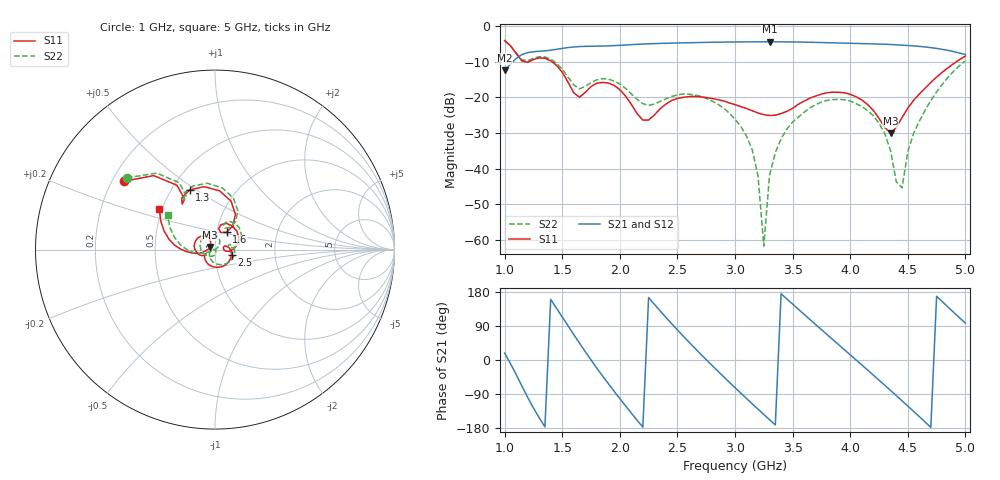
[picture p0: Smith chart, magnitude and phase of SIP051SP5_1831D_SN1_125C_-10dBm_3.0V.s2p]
# GHz  S  dB  R  50
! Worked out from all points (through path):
!   81 points, 1 GHz to 5 GHz, reference 50 ohm
!   highest |S21| = -4.32 dB at 3.3 GHz (marker M1); lowest = -12.4 dB at 1 GHz (marker M2)
!   lowest |S11| = -30.0 dB at 4.35 GHz (marker M3), VSWR 1.07, Z = 47.2 + j1.32 ohm
!   |S11| at or under -10 dB: 1.188 GHz to 1.206 GHz (18.48 MHz wide, 1.54 % of centre); 1.414 GHz to 4.919 GHz (3.506 GHz wide, 111 % of centre)
!   |S22| runs from -61.8 to -4.0 dB; largest |S21 - S12| = 0.0017
!   S11 on the Smith chart (normalised r, x): 1 GHz: 0.25, +0.31; 1.3 GHz: 0.62, +0.47; 1.6 GHz: 1.11, +0.22; 2.5 GHz: 1.20, -0.07; 5 GHz: 0.48, +0.25
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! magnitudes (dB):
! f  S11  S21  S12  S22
! 1 GHz  -4.0  -12.4  -12.4  -4.0
! 1.3 GHz  -8.8  -7.0  -7.0  -8.5
! 1.6 GHz  -18.7  -5.8  -5.8  -16.5
! 1.7 GHz  -18.6  -5.6  -5.6  -16.9
! 1.95 GHz  -16.6  -5.4  -5.4  -15.4
! 2.2 GHz  -26.4  -5.0  -5.0  -21.7
! 2.35 GHz  -23.2  -4.8  -4.8  -21.1
! 2.5 GHz  -20.3  -4.7  -4.7  -19.3
! 3 GHz  -22.0  -4.4  -4.4  -26.1
! 3.15 GHz  -23.7  -4.3  -4.3  -34.8
! 3.2 GHz  -24.4  -4.3  -4.3  -42.1
! 3.25 GHz  -24.8  -4.3  -4.3  -61.8
! 3.3 GHz  -25.1  -4.3  -4.3  -41.8
! 3.45 GHz  -23.9  -4.4  -4.3  -28.9
! 3.7 GHz  -19.6  -4.5  -4.5  -22.0
! 4.1 GHz  -20.7  -4.8  -4.8  -22.5
! 4.35 GHz  -30.0  -5.1  -5.1  -34.9
! 4.4 GHz  -28.4  -5.2  -5.2  -43.7
! 4.45 GHz  -25.7  -5.3  -5.3  -45.5
! 4.5 GHz  -23.0  -5.4  -5.4  -35.2
! 4.6 GHz  -19.0  -5.6  -5.6  -26.7
! 5 GHz  -8.3  -7.9  -7.9  -9.7
